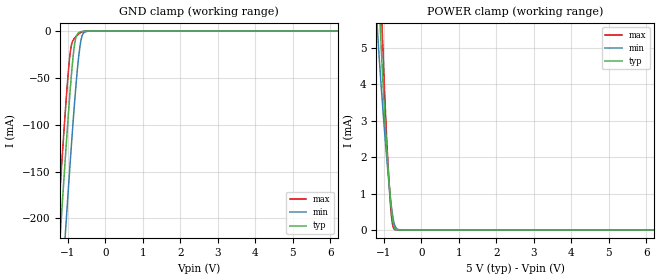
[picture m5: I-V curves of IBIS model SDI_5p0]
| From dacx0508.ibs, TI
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|   Model
[Model]   SDI_5p0
Model_type   Input
Vinl = 1.5
Vinh = 3.5
|   typ   min   max
C_comp   1.0511pF   0.96748pF   1.07561pF
| Where nom  PVT is Nominal Process, 5.0V, 27C
|   Fast PVT is Strong Process,  5.5V, -40C
|   Slow PVT is Weak Process,   4.5V, 125C
[Voltage Range]   5   4.5   5.5
|Junction Temperature
[Temperature Range]   27   125   -40
[Power Clamp Reference]   5   4.5   5.5
[GND Clamp Reference]   0   0   0
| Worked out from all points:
|   GND clamp passes 1 mA (typ) near -0.68 V on its own axis
|   POWER clamp passes 1 mA (typ) near -0.84 V on its own axis
[GND Clamp]
|   Voltage   I(typ)   I(min)   I(max)
-5V       -2.703A    -2.778A    -2.657A
-1.43V    -358.5mA   -440.6mA   -306.7mA
-1.25V    -245.1mA   -327.4mA   -193.3mA
-1.13V    -171.5mA   -253.3mA   -120.3mA
-1.085V   -144.5mA   -225.9mA   -94.03mA
-1.04V    -118.1mA   -198.9mA   -68.97mA
-935mV    -60.33mA   -137.4mA   -21.84mA
-815mV    -12.18mA   -72.18mA   -7.086mA
-665mV    -777.3uA   -12.57mA   -1.674mA
-575mV    -125.7uA   -1.55mA    -325.7uA
-455mV    -5.87uA    -57.8uA    -8.766uA
10V       0A         0A         0A
[POWER Clamp]
|   Voltage   I(typ)   I(min)   I(max)
-5V       112.6mA    89.62mA    135.5mA
-1.25V    9.313mA    6.889mA    11.73mA
-1.16V    7.09mA     5.323mA    8.952mA
-1.085V   5.353mA    4.164mA    6.71mA
-1.055V   4.705mA    3.732mA    5.844mA
-1.04V    4.395mA    3.522mA    5.421mA
-935mV    2.473mA    2.136mA    2.756mA
-875mV    1.537mA    1.42mA     1.551mA
-830mV    923.1uA    940.4uA    805uA
-770mV    311.4uA    429uA      163.5uA
-695mV    30.69uA    91.82uA    5.646uA
10V       0A         0A         0A
